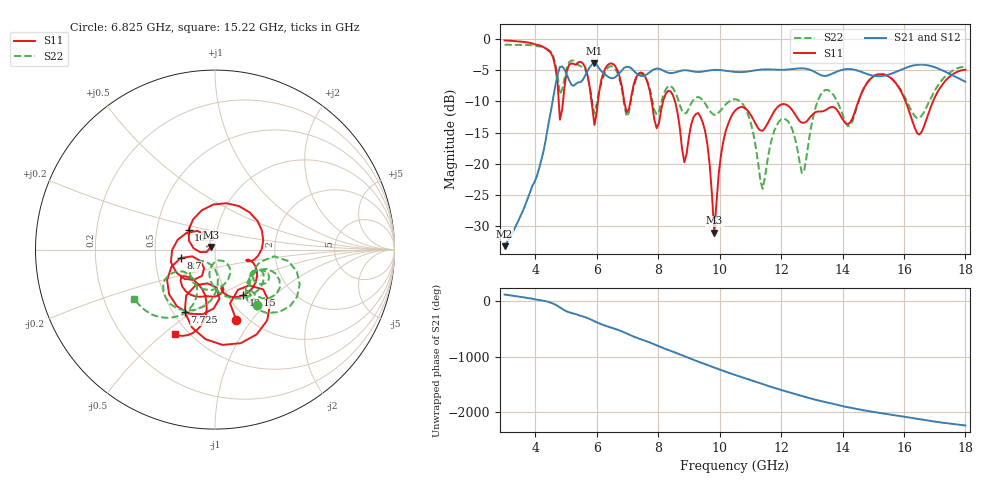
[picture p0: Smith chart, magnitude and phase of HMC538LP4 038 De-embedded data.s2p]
! Chelmsford, MA 01824
! http://www.hittite.com
! Tel: 978-250-3343
! Fax: 978-250-3373
! Device  :  HMC538LP4
! Description:  600 Analog Phase Shifter
! Frequency  :  6.0 GHz - 15.0 GHz
! Package  :  LP4  - 4x4 mm Quad Flatpack No-Lead (QFN) Plastic Package: 24 pin
! Ports  :  2 RF, 1 DC
!  Pin  3  = Rfin  = Port 1
!  Pin  16  = Rfout = Port 2
!  pin  21  = vCTL
! Voltages:  VCTL  = 0 to 5.0 Volts
! Currents :  Vb(V)  Vd(V)  Ib(mA)  Id(mA)
!  0.00  3.80  0.000000	0.475424
! Data:  The device was measured on evaluation board 111296-1.
!  Data was collected using a calibrated network analyzer.
!  The evaluation circuit board was modeled and simulated.This was use
!  to removed the evaluation board circuit from the measured data.
!  The reference plane is the center of the package pin.
! Misc:  Lot #
!Date Measured:  03 - 11 -2009
! Date:  03 - 17 -2009
! Note:
!  Hittite Microwave supplies this data as a sample of measured data at the
!  package pin for this package product.  Your particular data for this product
!  may vary.
!  Data was taken at 25 degrees C.
!  Hittite Microwave reserves the right to change this data at anytime.
# MHz S MA R 50
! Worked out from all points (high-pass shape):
!   201 points, 3 GHz to 18 GHz, reference 50 ohm
!   highest |S21| = -3.87 dB at 5.925 GHz (marker M1); lowest = -33.3 dB at 3 GHz (marker M2)
!   |S21| within 3 dB of the highest: 4.676 GHz to 5.131 GHz (454.9 MHz wide, 9.28 % of centre); 5.477 GHz to end of sweep
!   lowest |S11| = -31.1 dB at 9.825 GHz (marker M3), VSWR 1.06, Z = 47.6 + j1.37 ohm
!   |S11| at or under -10 dB: 7.786 GHz to 8.16 GHz (373.5 MHz wide, 4.68 % of centre); 8.549 GHz to 14.51 GHz (5.966 GHz wide, 51.7 % of centre); 16.05 GHz to 16.95 GHz (893.5 MHz wide, 5.42 % of centre)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
!   |S22| runs from -24.1 to -0.9 dB; largest |S21 - S12| = 0.0028
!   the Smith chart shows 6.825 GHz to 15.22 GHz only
!   S11 on the Smith chart (normalised r, x): 6.825 GHz: 0.90, -0.84; 7.725 GHz: 0.57, -0.47; 8.7 GHz: 0.68, -0.07; 10.2 GHz: 0.73, +0.16; 12.15 GHz: 1.18, -0.66; 15.22 GHz: 0.42, -0.55
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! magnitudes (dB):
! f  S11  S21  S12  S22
! 3 GHz  -0.2  -33.3  -33.2  -0.9
! 4.5 GHz  -2.1  -11.7  -11.8  -2.0
! 4.8 GHz  -12.9  -4.4  -4.4  -8.9
! 5.55 GHz  -3.9  -6.5  -6.5  -4.5
! 5.925 GHz  -13.8  -3.9  -3.9  -12.0
! 6.3 GHz  -4.5  -5.8  -5.8  -5.0
! 6.825 GHz  -7.8  -4.9  -4.9  -8.3
! 7.725 GHz  -8.3  -5.3  -5.3  -8.0
! 8.025 GHz  -13.5  -4.7  -4.7  -11.6
! 8.7 GHz  -14.1  -5.1  -5.1  -10.5
! 9.45 GHz  -13.4  -5.2  -5.2  -9.8
! 9.825 GHz  -31.1  -4.9  -4.9  -12.2
! 10.2 GHz  -14.7  -5.1  -5.1  -10.5
! 10.5 GHz  -11.5  -5.2  -5.3  -9.6
! 11.4 GHz  -14.7  -4.9  -4.9  -24.1
! 12.15 GHz  -10.5  -4.9  -4.9  -12.9
! 12.68 GHz  -13.4  -4.7  -4.7  -21.5
! 13.05 GHz  -12.0  -5.1  -5.1  -12.4
! 15.22 GHz  -5.6  -5.9  -6.0  -5.6
! 15.53 GHz  -6.1  -5.7  -5.7  -6.0
! 16.5 GHz  -15.3  -4.1  -4.1  -12.7
! 18 GHz  -4.9  -6.8  -6.8  -4.4
